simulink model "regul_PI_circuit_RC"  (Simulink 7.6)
settings: Solver=ode15s  StartTime=0.0  StopTime=N  RelTol=1e-3
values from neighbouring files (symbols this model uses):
  R = 4    [parametres.m]    (also in Prog_callbacks.m = 1000; oscillateur_dephasage.m = 1000; Calcul_Ampl_phase_A.m = 1; circuit_RLC_parallele_.m)
undefined symbols (not defined in the file or in its folder): R_Integ
libraries: fl_lib x16, nesl_utility x3

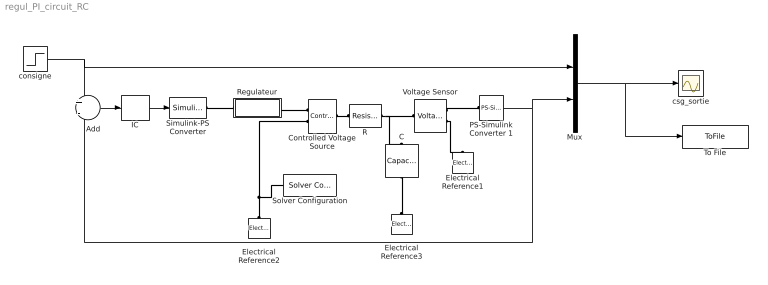
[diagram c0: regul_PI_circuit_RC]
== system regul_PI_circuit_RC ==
  Add : Sum  Inputs=+-
  C : fl_lib/Electrical/Electrical Elements/Capacitor  DialogController=NetworkEngine.DynNeDlgSource  SystemSampleTime=-1  c=C F  v0=0 V  r=1e-6 Ohm  g=0 1/Ohm  i_Log=off  v_Log=off  vc_Log=off  LocalVarNames=|current|voltage|power  LocalVarDescs=|Capacitor current (A)|Voltage across capacitor (V)|Power (W)  LocalVarLogging=[0 0 0]
  Controlled Voltage Source : fl_lib/Electrical/Electrical Sources/Controlled Voltage Source  DialogController=NetworkEngine.DynNeDlgSource  SystemSampleTime=-1  i_Log=off  v_Log=off  LocalVarNames=|current|voltage|power  LocalVarDescs=|Current (A)|Voltage (V)|Power (W)  LocalVarLogging=[0 0 0]
  Electrical Reference1 : fl_lib/Electrical/Electrical Elements/Electrical Reference  DialogController=NetworkEngine.DynNeDlgSource  SystemSampleTime=-1  i_Log=off  LocalVarNames=|i  LocalVarDescs=|i  LocalVarLogging=[]
  Electrical Reference2 : fl_lib/Electrical/Electrical Elements/Electrical Reference  DialogController=NetworkEngine.DynNeDlgSource  SystemSampleTime=-1  i_Log=off  LocalVarNames=|i  LocalVarDescs=|i  LocalVarLogging=[]
  Electrical Reference3 : fl_lib/Electrical/Electrical Elements/Electrical Reference  DialogController=NetworkEngine.DynNeDlgSource  SystemSampleTime=-1  i_Log=off  LocalVarNames=|i  LocalVarDescs=|i  LocalVarLogging=[]
  IC : InitialCondition  Value=0
  Mux : Mux  Inputs=2
  PS-Simulink Converter 1 : nesl_utility/PS-Simulink Converter  DialogController=NetworkEngine.DynNeUtilDlgSource  SystemSampleTime=-1  PhysicalDomain=network_engine_domain  LeftPortType=input  RightPortType=output  SubClassName=ps_output  Unit=1  AffineConversion=off
  R : fl_lib/Electrical/Electrical Elements/Resistor  DialogController=NetworkEngine.DynNeDlgSource  SystemSampleTime=-1  R=R Ohm  i_Log=off  v_Log=off  LocalVarNames=|current|voltage|power  LocalVarDescs=|Resistor current (A)|Voltage across resistor (V)|Power (W)  LocalVarLogging=[0 0 0]
  Regulateur : Subsystem  InitFcn=R_Integ=1e2;C_Integ=5e-4;R=1e3;C=1e-3;N=50;
  Simulink-PS Converter : nesl_utility/Simulink-PS Converter  DialogController=NetworkEngine.DynNeUtilDlgSource  SystemSampleTime=-1  PhysicalDomain=network_engine_domain  LeftPortType=input  RightPortType=output  SubClassName=ps_input  Unit=1  AffineConversion=off  InputFilterTimeConstant=.001  UdotUserProvided=0
  Solver Configuration : nesl_utility/Solver Configuration  DialogController=NetworkEngine.DynNeUtilDlgSource  SystemSampleTime=-1  PhysicalDomain=network_engine_domain  LeftPortType=input  RightPortType=generic  SubClassName=solver  Accelerate=off  Profile=off  ResidualTolerance=1e-9  MaxNonlinIter=12  MaxModeIter=2  DoFixedCost=off  UseLocalSampling=off  DoDC=off  LinearAlgebra=Sparse  LocalSolverSampleTime=.001  LocalSolverChoice=NE_BACKWARD_EULER_ADVANCER  UseLocalSolver=off
  To File : ToFile  Filename=cons_rep.mat  MatrixName=x
  Voltage Sensor : fl_lib/Electrical/Electrical Sensors/Voltage Sensor  DialogController=NetworkEngine.DynNeDlgSource  SystemSampleTime=-1  i1_Log=off  v1_Log=off  LocalVarNames=|i1|v1  LocalVarDescs=|i1|v1  LocalVarLogging=[]
  consigne : Step  Time=5  After=5  SampleTime=0
  csg_sortie : Scope
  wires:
  consigne/1 -> Mux/1, Add/1
  PS-Simulink Converter 1/1 -> Mux/2, Add/2
  Mux/1 -> csg_sortie/1, To File/1
  Add/1 -> IC/1
  IC/1 -> Simulink-PS Converter/1
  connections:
  Voltage Sensor/RConn2 -- Electrical Reference1/LConn1
  Voltage Sensor/RConn1 -- PS-Simulink Converter 1/LConn1
  Controlled Voltage Source/LConn1 -- R/LConn1
  Electrical Reference2/LConn1 -- Controlled Voltage Source/RConn2 -- Solver Configuration/RConn1
  Regulateur/RConn1 -- Controlled Voltage Source/RConn1
  Simulink-PS Converter/RConn1 -- Regulateur/LConn1
  C/RConn1 -- Electrical Reference3/LConn1
  R/RConn1 -- C/LConn1 -- Voltage Sensor/LConn1

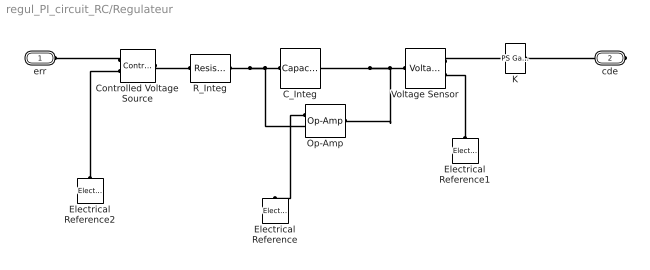
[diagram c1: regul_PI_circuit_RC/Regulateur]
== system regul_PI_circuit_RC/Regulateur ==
  C_Integ : fl_lib/Electrical/Electrical Elements/Capacitor  DialogController=NetworkEngine.DynNeDlgSource  SystemSampleTime=-1  c=C_Integ F  v0=0 V  r=1e-12 Ohm  g=0 1/Ohm  i_Log=off  v_Log=off  vc_Log=off  LocalVarNames=|current|voltage|power  LocalVarDescs=|Capacitor current (A)|Voltage across capacitor (V)|Power (W)  LocalVarLogging=[0 0 0]
  Controlled Voltage Source : fl_lib/Electrical/Electrical Sources/Controlled Voltage Source  DialogController=NetworkEngine.DynNeDlgSource  SystemSampleTime=-1  i_Log=off  v_Log=off  LocalVarNames=|current|voltage|power  LocalVarDescs=|Current (A)|Voltage (V)|Power (W)  LocalVarLogging=[0 0 0]
  Electrical Reference : fl_lib/Electrical/Electrical Elements/Electrical Reference  DialogController=NetworkEngine.DynNeDlgSource  SystemSampleTime=-1  i_Log=off  LocalVarNames=|i  LocalVarDescs=|i  LocalVarLogging=[]
  Electrical Reference1 : fl_lib/Electrical/Electrical Elements/Electrical Reference  DialogController=NetworkEngine.DynNeDlgSource  SystemSampleTime=-1  i_Log=off  LocalVarNames=|i  LocalVarDescs=|i  LocalVarLogging=[]
  Electrical Reference2 : fl_lib/Electrical/Electrical Elements/Electrical Reference  DialogController=NetworkEngine.DynNeDlgSource  SystemSampleTime=-1  i_Log=off  LocalVarNames=|i  LocalVarDescs=|i  LocalVarLogging=[]
  K : fl_lib/Physical Signals/Functions/PS Gain  DialogController=NetworkEngine.DynNeDlgSource  SystemSampleTime=-1  gain=-0.02  LocalVarLogging=[]
  Op-Amp : fl_lib/Electrical/Electrical Elements/Op-Amp  DialogController=NetworkEngine.DynNeDlgSource  SystemSampleTime=-1  i1_Log=off  v1_Log=off  outI_Log=off  LocalVarNames=|i1|v1|outI  LocalVarDescs=|i1|v1|outI  LocalVarLogging=[]
  R_Integ : fl_lib/Electrical/Electrical Elements/Resistor  DialogController=NetworkEngine.DynNeDlgSource  SystemSampleTime=-1  R=R_Integ Ohm  i_Log=off  v_Log=off  LocalVarNames=|current|voltage|power  LocalVarDescs=|Resistor current (A)|Voltage across resistor (V)|Power (W)  LocalVarLogging=[0 0 0]
  Voltage Sensor : fl_lib/Electrical/Electrical Sensors/Voltage Sensor  DialogController=NetworkEngine.DynNeDlgSource  SystemSampleTime=-1  i1_Log=off  v1_Log=off  LocalVarNames=|i1|v1  LocalVarDescs=|i1|v1  LocalVarLogging=[]
  err : PMIOPort  Port=1  Side=Left
  cde : PMIOPort  Port=2  Side=Right
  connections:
  Voltage Sensor/RConn1 -- K/LConn1
  Controlled Voltage Source/RConn1 -- err/RConn1
  cde/RConn1 -- K/RConn1
  Voltage Sensor/LConn1 -- Op-Amp/RConn1 -- C_Integ/RConn1
  Electrical Reference1/LConn1 -- Voltage Sensor/RConn2
  Op-Amp/LConn1 -- Electrical Reference/LConn1
  Electrical Reference2/LConn1 -- Controlled Voltage Source/RConn2
  C_Integ/LConn1 -- Op-Amp/LConn2 -- R_Integ/RConn1
  Controlled Voltage Source/LConn1 -- R_Integ/LConn1
